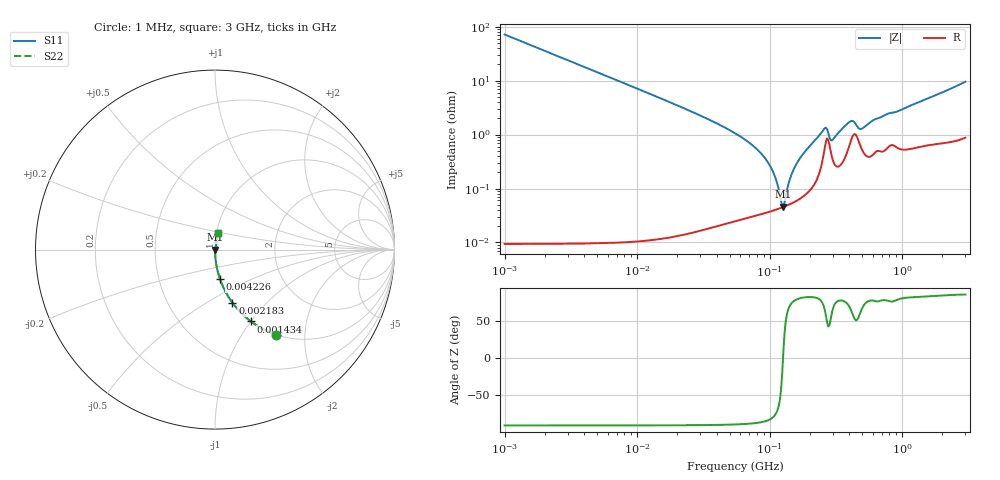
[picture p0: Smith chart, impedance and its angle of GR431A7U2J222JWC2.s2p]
!Murata Part Number: GR431A7U2J222JWC2
!These Parameters are Measured in Series Mode Connection
!Data Generated on Jun 10, 2025
!  o--ll--o
!Port1  Port2
!  o------o
!Operation Temp=25[degC], DC Bias Voltage=0[V]
!Freq. Start=1000[kHz] Stop=3[GHz] 401[Steps]
# Hz S RI R 50
!Freq.(Hz) S11(Real) S11(Imag) S21(Real) S21(Imag) S12(Real) S12(Imag) S22(Real) S22(Imag)
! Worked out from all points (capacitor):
!   401 points, 1 MHz to 3 GHz, reference 50 ohm
!   read as one part in series: C = 2.22 nF near 1.041 MHz
!   lowest |Z| = 46 mohm at 127 MHz (marker M1)
!   series resonance near 126.2 MHz, so ESL is about 720 pH
!   S11 on the Smith chart (normalised r, x): 1 MHz: 1.00, -1.43; 1.434 MHz: 1.00, -1.00; 2.183 MHz: 1.00, -0.66; 4.226 MHz: 1.00, -0.34; 3 GHz: 1.02, +0.19
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1000000  0.3396 -0.4735  0.6604 0.4735  0.6604 0.4735  0.3396 -0.4735
1433740  0.2001 -0.4  0.7999 0.4  0.7999 0.4  0.2001 -0.4
2182827  0.0974 -0.2964  0.9026 0.2964  0.9026 0.2964  0.0974 -0.2964
3823119  0.034 -0.181  0.966 0.181  0.966 0.181  0.034 -0.181
4225536  0.028 -0.1648  0.972 0.1648  0.972 0.1648  0.028 -0.1648
1.461624e7  0.00245 -0.0482  0.9976 0.0482  0.9976 0.0482  0.00245 -0.0482
5.477226e7  0.000359 -0.0106  0.9996 0.0106  0.9996 0.0106  0.000359 -0.0106
7.544761e7  0.000342 -0.00611  0.9997 0.00611  0.9997 0.00611  0.000342 -0.00611
9.402997e7  0.000367 -0.00341  0.9996 0.00341  0.9996 0.00341  0.000367 -0.00341
1.081723e8  0.000398 -0.00178  0.9996 0.00178  0.9996 0.00178  0.000398 -0.00178
1.219755e8  0.000438 -0.000393  0.9996 0.000393  0.9996 0.000393  0.000438 -0.000393
1.269575e8  0.000455 6.97e-05  0.9995 -6.97e-05  0.9995 -6.97e-05  0.000455 6.97e-05
1.295243e8  0.000464 0.000302  0.9995 -0.000302  0.9995 -0.000302  0.000464 0.000302
1.431579e8  0.000518 0.00148  0.9995 -0.00148  0.9995 -0.00148  0.000518 0.00148
1.550909e8  0.000575 0.00246  0.9994 -0.00246  0.9994 -0.00246  0.000575 0.00246
2.094008e8  0.00108 0.00677  0.9989 -0.00677  0.9989 -0.00677  0.00108 0.00677
2.609752e8  0.00591 0.0117  0.9941 -0.0117  0.9941 -0.0117  0.00591 0.0117
3.002264e8  0.00336 0.00732  0.9966 -0.00732  0.9966 -0.00732  0.00336 0.00732
4.0536e8  0.00721 0.0158  0.9928 -0.0158  0.9928 -0.0158  0.00721 0.0158
4.951867e8  0.00549 0.0115  0.9945 -0.0115  0.9945 -0.0115  0.00549 0.0115
8.005644e8  0.00662 0.0238  0.9934 -0.0238  0.9934 -0.0238  0.00662 0.0238
3e9  0.0174 0.0925  0.9826 -0.0925  0.9826 -0.0925  0.0174 0.0925
